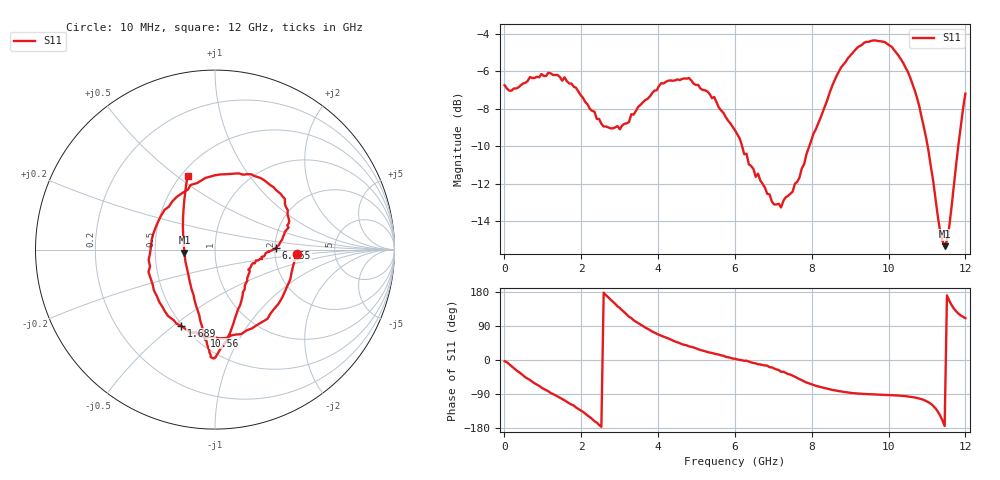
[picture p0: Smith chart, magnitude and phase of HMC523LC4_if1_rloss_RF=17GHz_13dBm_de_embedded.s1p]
!Hittite Microwave Corporation
!20 Alpha Rd
!Chelmsford, MA 01824
!Tel: 978-250-3343
!Fax: 978-250-3373
!Device: HMC523LC4, 0.01-12 GHz, GaAs MMIC Double-Balanced Mixer
!Misc: IF1 Return Loss with RF=17GHz at 13 dBm, Room
# MHZ S MA R 50
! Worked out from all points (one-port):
!   201 points, 10 MHz to 12 GHz, reference 50 ohm
!   lowest |S11| = -15.3 dB at 11.46 GHz (marker M1), VSWR 1.41, Z = 35.4 - j1.27 ohm
!   |S11| at or under -10 dB: 6.191 GHz to 7.939 GHz (1.748 GHz wide, 24.7 % of centre); 11.02 GHz to 11.81 GHz (796.2 MHz wide, 6.97 % of centre)
!   S11 on the Smith chart (normalised r, x): 10 MHz: 2.69, -0.16; 1.689 GHz: 0.49, -0.53; 6.065 GHz: 2.03, +0.04; 10.56 GHz: 0.57, -0.71; 12 GHz: 0.54, +0.55
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10  0.46 -3.0
429.65  0.46 -35.4
789.35  0.481 -61.5
1149.05  0.497 -82.7
1508.75  0.473 -103.0
1688.6  0.465 -114.1
2348.05  0.391 -161.5
2707.75  0.355 165.6
3007.5  0.351 137.1
3307.25  0.385 110.7
3666.95  0.42 85.8
4086.6  0.466 64.1
4506.25  0.477 46.8
5285.6  0.443 21.0
6005  0.349 3.3
6064.95  0.34 1.4
7024.15  0.221 -22.4
7503.75  0.239 -41.3
8582.85  0.471 -79.8
9002.5  0.552 -86.7
9841.8  0.602 -91.8
10501.25  0.5 -96.4
10561.2  0.483 -97.1
11040.8  0.307 -111.6
11340.55  0.188 -146.3
11460.45  0.171 -174.2
11580.35  0.193 156.6
12000  0.437 110.4
